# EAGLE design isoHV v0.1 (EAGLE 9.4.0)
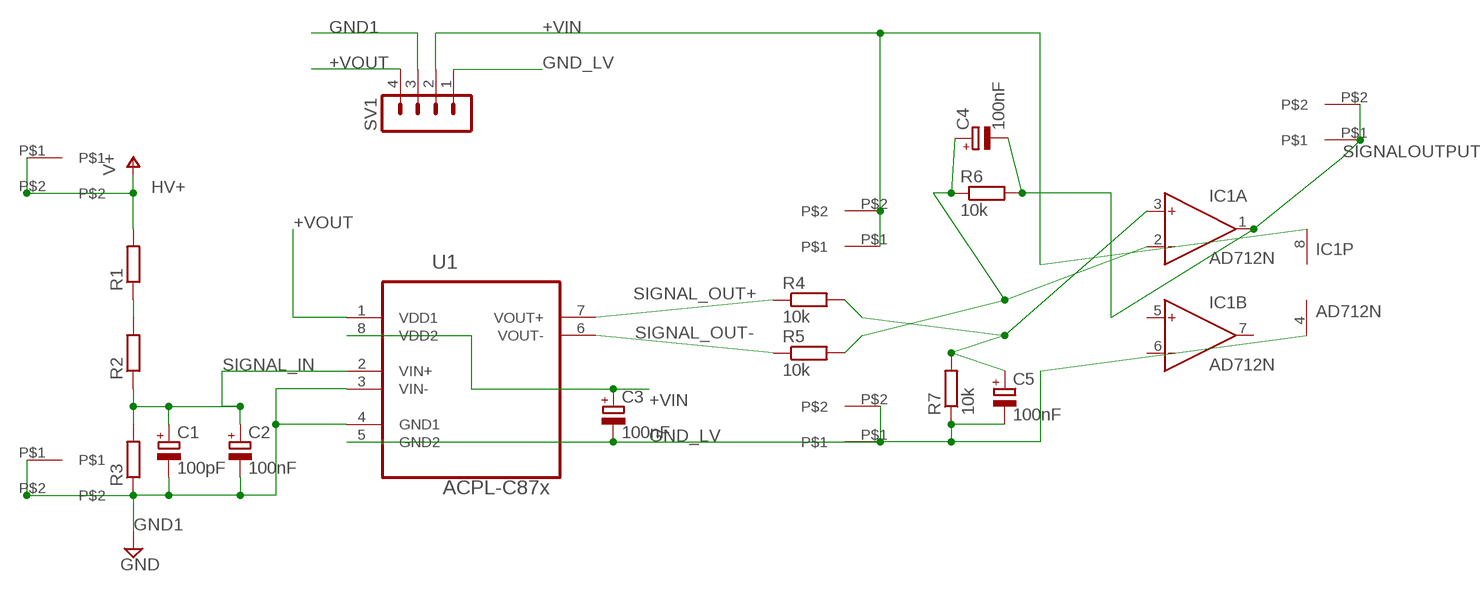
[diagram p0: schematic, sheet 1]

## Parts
C1  100pF  CPOL-EUB45181A  [B45181A]
C2  100nF  CPOL-EUB45181A  [B45181A]
C3  100nF  CPOL-EUB45181A  [B45181A]
C4  100nF  CPOL-EUB45181A  [B45181A]
C5  100nF  CPOL-EUB45181A  [B45181A]
IC1  AD712N  [DIL08]
R1  R-EU_0411/15  [0411/15]
R2  R-EU_0411/15  [0411/15]
R3  R-EU_0411/15  [0411/15]
R4  10k  R-EU_0204/7  [0204/7]
R5  10k  R-EU_0204/7  [0204/7]
R6  10k  R-EU_0204/7  [0204/7]
R7  10k  R-EU_0204/7  [0204/7]
SV1  MA04-1  [MA04-1]
U1  ACPL-C87x  ACPL-C79B-000E  [SOIC127P1150X330-8N]
U$1  7.62MM_TERMINAL_BLOCK  [7.62MM]
U$2  7.62MM_TERMINAL_BLOCK  [7.62MM]
U$3  7.62MM_TERMINAL_BLOCK  [7.62MM]
U$4  7.62MM_TERMINAL_BLOCK  [7.62MM]
U$5  7.62MM_TERMINAL_BLOCK  [7.62MM]

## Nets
+VIN: C3.+ IC1.8(P:V+) SV1.2 U1.8(VDD2) U$3.P$1 U$3.P$2
+VOUT: SV1.4 U1.1(VDD1)
GND1: C1.- C2.- R3.1 SV1.3 U1.3(VIN-) U1.4(GND1) U$2.P$1 U$2.P$2 ; supply symbol labelled GND
GND_LV: C3.- C5.- IC1.4(P:V-) R7.1 SV1.1 U1.5(GND2) U$4.P$1 U$4.P$2
HV+: R1.2 U$1.P$1 U$1.P$2 ; supply symbol labelled V+
N$1: C5.+ IC1.3(A:IN+) R4.2 R7.2
N$2: R1.1 R2.2
N$5: C4.+ IC1.2(A:IN-) R5.2 R6.1
SIGNAL_IN: C1.+ C2.+ R2.1 R3.2 U1.2(VIN+)
SIGNAL_OUT+: R4.1 U1.7(VOUT+)
SIGNAL_OUT-: R5.1 U1.6(VOUT-)
SIGNALOUTPUT: C4.- IC1.1(A:OUT) R6.2 U$5.P$1 U$5.P$2
Unconnected: IC1.5(B:IN+) IC1.6(B:IN-) IC1.7(B:OUT)

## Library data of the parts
C1-C5 = rcl:CPOL-EU: POLARIZED CAPACITOR, European symbol; SPICEPREFIX: C
IC1 = analog-devices:AD712: Dual Precision, Low Cost, High Speed BiFET Op Amp Source: http://www.analog.com/static/imported-files/data_sheets/AD712.pdf; MF: ALTERA CORPORATION; MPN: AD712JNZ; OC_FARNELL: 9604898; OC_NEWARK: 59K4554
R1-R7 = rcl:R-EU_: RESISTOR, European symbol; SPICEPREFIX: R
SV1 = con-lstb:MA04-1: PIN HEADER; OC_FARNELL: unknown; OC_NEWARK: unknown
U1 = Avago_By_element14_Batch_1:ACPL-C79B-000E: Precision Miniature Isolation Amplifiers; DESCRIPTION: Precision Miniature Isolation Amplifiers; MPN: ACPL-C79B-000E; OC_FARNELL: 1854253; OC_NEWARK: 74R5803; PACKAGE: SOIC-8; SUPPLIER: AVAGO TECHNOLOGIES
U$1-U$5 = 7.62mm terminal block:7.62MM_TERMINAL_BLOCK

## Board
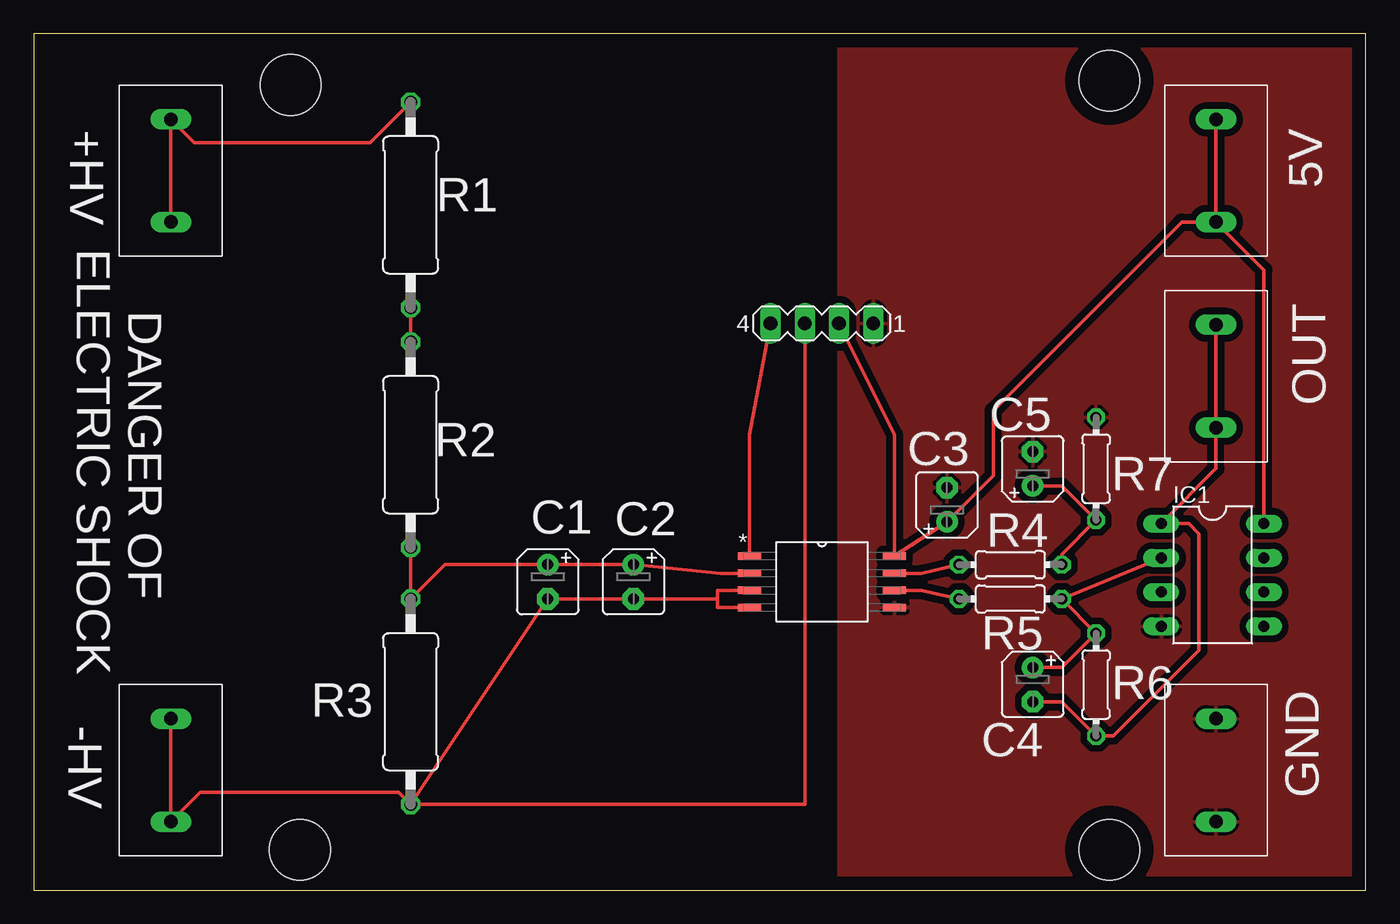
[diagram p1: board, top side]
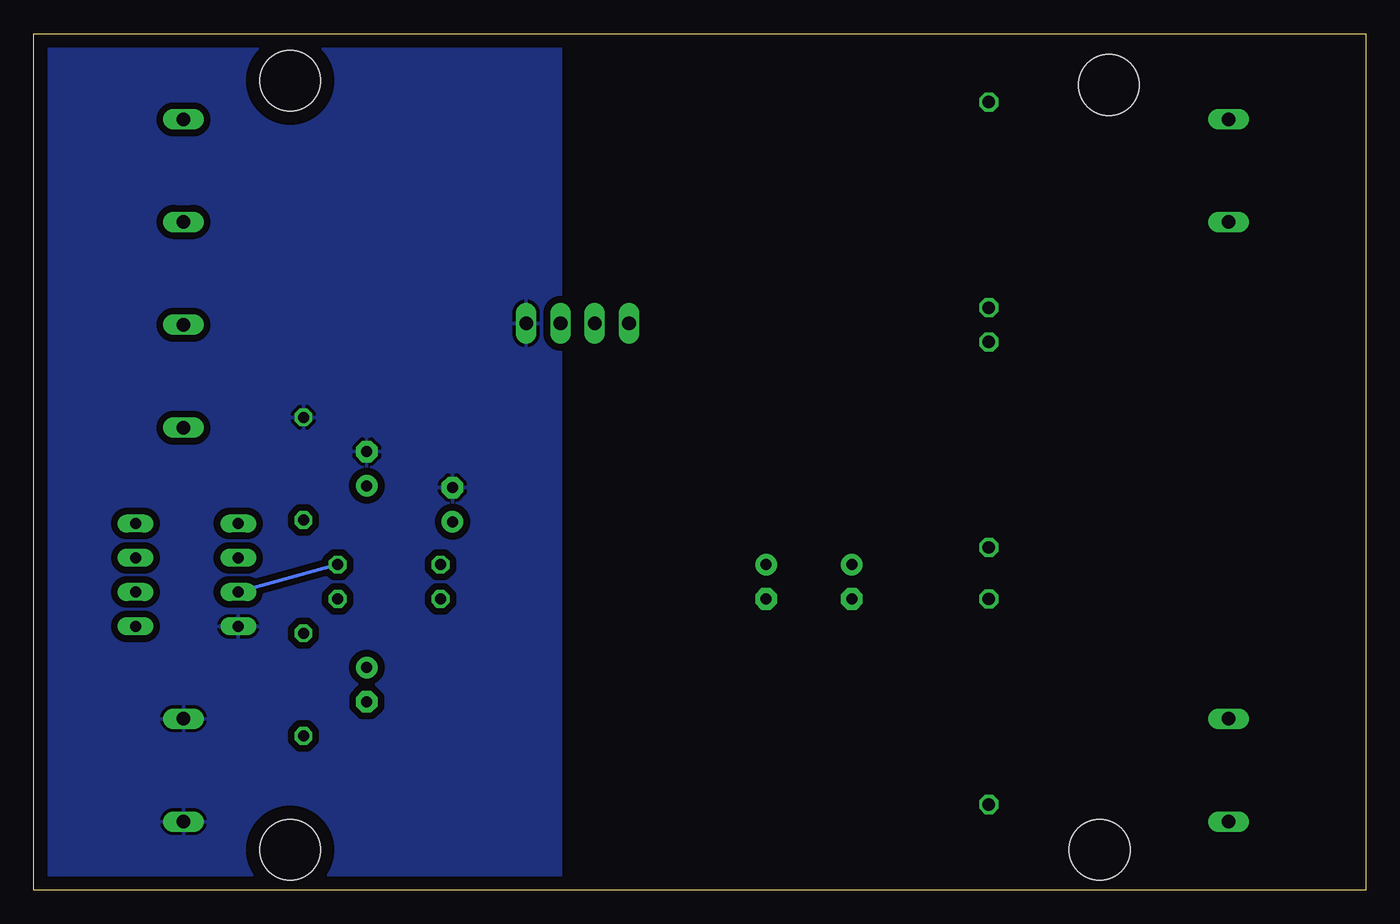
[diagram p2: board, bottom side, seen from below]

Size 98.73 x 63.49 mm. Coordinates in mm from the lower left corner, seen from the top.
Outline: 0,0 98.73,0 98.73,63.49 0,63.49 0,0
Copper layers (1*16): Top 0.035mm / dielectric 0.15mm / Bottom 0.035mm
Design rules "default": minimum track width 6mil, minimum drill 0.35mm, track to track 6mil, track to pad 6mil, pad to pad 6mil, via to via 6mil, smd to smd 6mil, copper to edge 40mil, drill to drill 6mil, minimum pad ring 10mil, minimum via ring 8mil, stop-mask expansion 4mil, vias tented up to drill 0mil, thermal gap 10mil
Holes 4.5 mm at 19.05,59.69 19.73,3 79.73,3 79.73,60

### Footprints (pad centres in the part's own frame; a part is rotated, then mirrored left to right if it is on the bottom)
B45181A = drill 0.813 pad 1.6: + -1.27,0 | drill 0.813 pad 1.6 octagon: - 1.27,0
DIL08 = drill 0.813 long: 1 -3.81,-3.81; 2 -1.27,-3.81; 3 1.27,-3.81; 4 3.81,-3.81; 5 3.81,3.81; 6 1.27,3.81; 7 -1.27,3.81; 8 -3.81,3.81
0411/15 = drill 0.914 octagon: 1 -7.62,0; 2 7.62,0
0204/7 = drill 0.813 octagon: 1 -3.81,0; 2 3.81,0
MA04-1 = drill 1.016 long: 1 -3.81,0; 2 -1.27,0; 3 1.27,0; 4 3.81,0
SOIC127P1150X330-8N = smd 1.702 x 0.559: 1 -5.385,1.905; 2 -5.385,0.635; 3 -5.385,-0.635; 4 -5.385,-1.905; 5 5.385,-1.905; 6 5.385,-0.635; 7 5.385,0.635; 8 5.385,1.905
7.62MM = drill 1 long: P$1 0,-3.81; P$2 0,3.81

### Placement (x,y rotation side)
C1  38.1,22.86 270 top
C2  44.45,22.86 270 top
C3  67.69,28.57 90 top
C4  74.04,15.24 270 top
C5  74.04,31.24 90 top
IC1  87.38,23.37 270 top
R1  27.94,50.8 90 top
R2  27.94,33.02 90 top
R3  27.94,13.97 90 top
R4  72.39,24.13 0 top
R5  72.39,21.59 0 top
R6  78.74,15.24 270 top
R7  78.74,31.24 270 top
SV1  58.42,42.02 180 top
U1  58.42,22.86 0 top
U$1  10.16,53.34 180 top
U$2  10.16,8.89 0 top
U$3  87.63,53.34 0 top
U$4  87.63,8.89 180 top
U$5  87.63,38.1 0 top

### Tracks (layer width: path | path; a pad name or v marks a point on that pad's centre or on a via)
+VIN
  Top 0.254: SV1.2 63.8,33.77 U1.8 C3.+ 71.12,30.73 71.12,35.56 85.09,49.53 U$3.P$1 | IC1.8 91.19,45.97 U$3.P$1 | U$3.P$2 U$3.P$1
+VOUT
  Top 0.254: SV1.4 53.03,33.77 U1.1
GND1
  Top 0.254: U1.3 50.67,22.23 50.67,21.59 | 50.67,21.59 50.67,20.95 U1.4 | U$2.P$2 U$2.P$1 12.32,7.24 27.05,7.24 R3.1 | R3.1 C1.- C2.- 50.67,21.59 | R3.1 57.15,6.35 SV1.3
GND_LV
  pour Top (isolate 0.508): 59.69,63.5 59.69,0 99.06,0 99.06,63.5
  pour Bottom (isolate 0.508): 99.06,63.5 99.06,0 59.69,0 59.69,63.5
HV+
  Top 0.254: U$1.P$2 U$1.P$1 11.89,55.42 24.94,55.42 R1.2
N$1
  Top 0.254: R4.2 76.2,24.89 R7.2 76.2,29.97 C5.+
  Bottom 0.254: R4.2 IC1.3
N$2
  Top 0.254: R1.1 R2.2
N$5
  Top 0.254: IC1.2 R5.2 R6.1 76.2,16.51 C4.+
SIGNAL_IN
  Top 0.254: R2.1 R3.2 30.48,24.13 C1.+ C2.+ 50.93,23.5 U1.2
SIGNAL_OUT+
  Top 0.254: U1.7 65.79,23.5 R4.1
SIGNAL_OUT-
  Top 0.254: U1.6 65.79,22.23 R5.1
SIGNALOUTPUT
  Top 0.254: U$5.P$2 U$5.P$1 87.63,31.24 IC1.1 85.6,27.18 86.36,26.42 86.36,17.78 80.01,11.43 R6.2 76.2,13.97 C4.-

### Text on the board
tNames: +HV | 5V | OUT | DANGER OF / ELECTRIC SHOCK | -HV | GND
